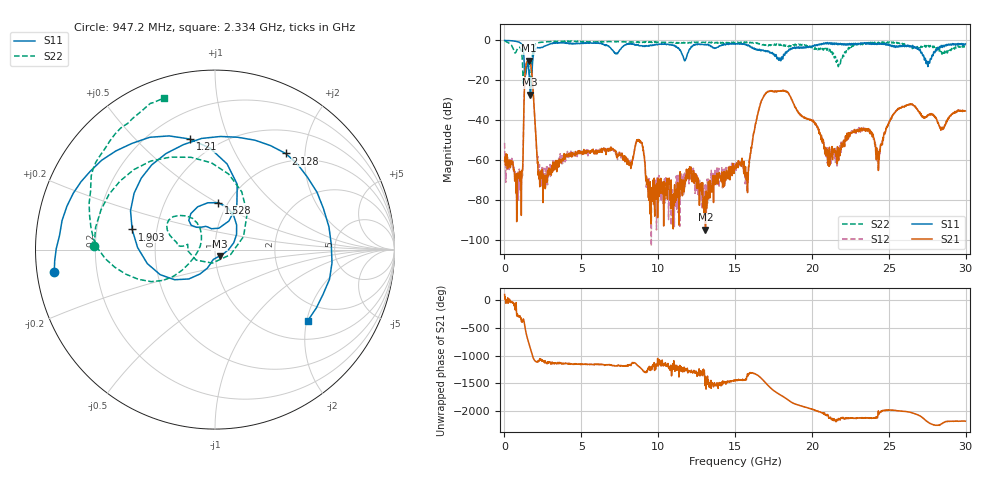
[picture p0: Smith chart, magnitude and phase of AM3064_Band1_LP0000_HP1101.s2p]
# Hz S DB R 50.0
!freq dBS11 angS11 dBS21 angS21 dBS12 angS12 dBS22 angS22
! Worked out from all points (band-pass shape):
!   1600 points, 10 MHz to 29.98 GHz, reference 50 ohm
!   highest |S21| = -10.15 dB at 1.584 GHz (marker M1); lowest = -94.6 dB at 13.07 GHz (marker M2)
!   |S21| within 3 dB of the highest: 1.382 GHz to 1.731 GHz (349.2 MHz wide, 22.4 % of centre)
!   lowest |S11| = -27.1 dB at 1.678 GHz (marker M3), VSWR 1.09, Z = 52.4 - j3.83 ohm
!   |S11| at or under -10 dB: 1.277 GHz to 1.841 GHz (563.8 MHz wide, 36.2 % of centre); 11.69951 GHz to 11.75666 GHz (57.15 MHz wide, 0.487 % of centre); 27.4 GHz to 27.68 GHz (282.9 MHz wide, 1.03 % of centre)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
!   |S22| runs from -22.3 to -0.2 dB; largest |S21 - S12| = 0.0053
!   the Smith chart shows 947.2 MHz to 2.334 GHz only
!   S11 on the Smith chart (normalised r, x): 947.2 MHz: 0.05, -0.07; 1.21 GHz: 0.36, +0.73; 1.528 GHz: 0.90, +0.51; 1.903 GHz: 0.36, +0.10; 2.128 GHz: 0.85, +1.64; 2.334 GHz: 1.47, -2.03
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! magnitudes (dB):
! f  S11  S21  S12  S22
! 10 MHz  -0.1  -60.5  -51.2  -0.2
! 947.2 MHz  -0.9  -68.4  -71.5  -3.4
! 1.21 GHz  -4.0  -58.1  -57.2  -20.8
! 1.528 GHz  -11.6  -10.2  -10.2  -10.6
! 1.584 GHz  -14.8  -10.2  -10.1  -13.4
! 1.678 GHz  -27.1  -11.2  -11.2  -21.5
! 1.903 GHz  -6.5  -30.1  -30.1  -3.7
! 2.128 GHz  -3.5  -59.0  -57.4  -1.5
! 2.334 GHz  -3.7  -67.6  -65.5  -1.0
! 5.015 GHz  -1.4  -55.8  -57.2  -0.7
! 8.745 GHz  -2.7  -50.2  -50.0  -1.1
! 10 GHz  -2.0  -68.9  -77.2  -0.9
! 13.07 GHz  -2.0  -94.6  -81.2  -1.0
! 15 GHz  -1.8  -63.6  -62.8  -1.3
! 15.81 GHz  -2.6  -76.1  -67.3  -1.2
! 17.12 GHz  -5.7  -25.8  -25.7  -2.5
! 19.99 GHz  -3.2  -40.1  -40.0  -3.5
! 21.13 GHz  -1.2  -53.4  -61.3  -4.5
! 23.36 GHz  -1.6  -44.4  -45.0  -1.8
! 24.3 GHz  -1.8  -58.6  -58.9  -0.9
! 25 GHz  -2.0  -41.5  -40.8  -1.1
! 29.98 GHz  -1.8  -35.3  -35.2  -3.1
